| IBIS file stm32f303x6x8_334_lqfp64.ibs
[IBIS ver] 4.2
[File name] stm32f303x6x8_334_lqfp64.ibs
[File Rev] 1
[Date]  29-09-2025
[Source] Data Created at STMicroelectronics
[Notes]  File originated from ELDO simulations.
[Disclaimer]  This information is for modeling purpose only and is
   not guaranted. The information is subject to change without
   notice.
[Copyright] Copyright 2025 STMicroelectronics Inc.
|   Component stm32f303x6x8_334_lqfp64
[Component] stm32f303x6x8_334_lqfp64
[Manufacturer] STMicroelectronics
[Package]
| variable   typ   min   max
R_pkg   0.0   0.0   0.0
L_pkg   0.0H   0.0H   0.0H
C_pkg   0.0F   0.0F   0.0F
[Pin]  signal_name   model_name   R_pin   L_pin   C_pin
1 VBAT POWER 68.980E-3 4.220E-9 120.000E-15
2 PC13 io8p_sudq_tc 63.756E-3 3.679E-9 93.469E-15
3 PC14-OSC32_IN io8p_sudq_tc 59.336E-3 3.221E-9 71.020E-15
4 PC15-OSC32_OUT io8p_sudq_tc 55.719E-3 2.846E-9 52.653E-15
5 PF0-OSC_IN io8p_wsudqh_i2c_ft 52.907E-3 2.555E-9 38.367E-15
6 PF1-OSC_OUT io8p_wsudqh_i2c_ft 50.897E-3 2.347E-9 28.163E-15
7 NRST ioreset_tc_v33 49.692E-3 2.222E-9 22.041E-15
8 PC0 io8p_sudq_tc 49.290E-3 2.180E-9 20.000E-15
9 PC1 io8p_sudq_tc 49.290E-3 2.180E-9 20.000E-15
10 PC2 io8p_sudq_tc 49.692E-3 2.222E-9 22.041E-15
11 PC3 io8p_sudq_tc 50.897E-3 2.347E-9 28.163E-15
12 VSSA GND 52.907E-3 2.555E-9 38.367E-15
13 VDDA POWER 55.719E-3 2.846E-9 52.653E-15
14 PA0 io8p_sudq_tc 59.336E-3 3.221E-9 71.020E-15
15 PA1 io8p_sudq_tc 63.756E-3 3.679E-9 93.469E-15
16 PA2 io8p_sudq_tc 68.980E-3 4.220E-9 120.000E-15
17 PA3 io8p_sudq_tc 68.980E-3 4.220E-9 120.000E-15
18 VSS GND 63.756E-3 3.679E-9 93.469E-15
19 VDD POWER 59.336E-3 3.221E-9 71.020E-15
20 PA4 io8p_sudq_tc 55.719E-3 2.846E-9 52.653E-15
21 PA5 io8p_sudq_tc 52.907E-3 2.555E-9 38.367E-15
22 PA6 io8p_sudq_tc 50.897E-3 2.347E-9 28.163E-15
23 PA7 io8p_sudq_tc 49.692E-3 2.222E-9 22.041E-15
24 PC4 io8p_sudq_tc 49.290E-3 2.180E-9 20.000E-15
25 PC5 io8p_sudq_tc 49.290E-3 2.180E-9 20.000E-15
26 PB0 io8p_sudq_tc 49.692E-3 2.222E-9 22.041E-15
27 PB1 io8p_sudq_tc 50.897E-3 2.347E-9 28.163E-15
28 PB2 io8p_sudq_tc 52.907E-3 2.555E-9 38.367E-15
29 PB10 io8p_sudq_tc 55.719E-3 2.846E-9 52.653E-15
30 PB11 io8p_sudq_tc 59.336E-3 3.221E-9 71.020E-15
31 VSS GND 63.756E-3 3.679E-9 93.469E-15
32 VDD POWER 68.980E-3 4.220E-9 120.000E-15
33 PB12 io8p_sudq_tc 68.980E-3 4.220E-9 120.000E-15
34 PB13 io8p_sudq_tc 63.756E-3 3.679E-9 93.469E-15
35 PB14 io8p_sudq_tc 59.336E-3 3.221E-9 71.020E-15
36 PB15 io8p_sudq_tc 55.719E-3 2.846E-9 52.653E-15
37 PC6 io8p_sudq_ft 52.907E-3 2.555E-9 38.367E-15
38 PC7 io8p_sudq_ft 50.897E-3 2.347E-9 28.163E-15
39 PC8 io8p_sudq_ft 49.692E-3 2.222E-9 22.041E-15
40 PC9 io8p_wsudqh_i2c_ft 49.290E-3 2.180E-9 20.000E-15
41 PA8 io8p_wsudqh_i2c_ft 49.290E-3 2.180E-9 20.000E-15
42 PA9 io8p_wsudqh_i2c_ft 49.692E-3 2.222E-9 22.041E-15
43 PA10 io8p_wsudqh_i2c_ft 50.897E-3 2.347E-9 28.163E-15
44 PA11 io8usb_lv_ft 52.907E-3 2.555E-9 38.367E-15
45 PA12 io8usb_lv_ft 55.719E-3 2.846E-9 52.653E-15
46 PA13 io8p_wsudqh_i2c_ft 59.336E-3 3.221E-9 71.020E-15
47 VSS GND 63.756E-3 3.679E-9 93.469E-15
48 VDD POWER 68.980E-3 4.220E-9 120.000E-15
49 PA14 io8p_wsudqh_i2c_ft 68.980E-3 4.220E-9 120.000E-15
50 PA15 io8p_wsudqh_i2c_ft 63.756E-3 3.679E-9 93.469E-15
51 PC10 io8p_sudq_ft 59.336E-3 3.221E-9 71.020E-15
52 PC11 io8p_sudq_ft 55.719E-3 2.846E-9 52.653E-15
53 PC12 io8p_sudq_ft 52.907E-3 2.555E-9 38.367E-15
54 PD2 io8p_sudq_ft 50.897E-3 2.347E-9 28.163E-15
55 PB3 io8p_sudq_ft 49.692E-3 2.222E-9 22.041E-15
56 PB4 io8p_sudq_ft 49.290E-3 2.180E-9 20.000E-15
57 PB5 io8p_wsudqh_i2c_ft 49.290E-3 2.180E-9 20.000E-15
58 PB6 io8p_wsudqh_i2c_ft 49.692E-3 2.222E-9 22.041E-15
59 PB7 io8p_wsudqh_i2c_ft 50.897E-3 2.347E-9 28.163E-15
60 BOOT0 vpp_test_hv 52.907E-3 2.555E-9 38.367E-15
61 PB8 io8p_wsudqh_i2c_ft 55.719E-3 2.846E-9 52.653E-15
62 PB9 io8p_wsudqh_i2c_ft 59.336E-3 3.221E-9 71.020E-15
63 VSS GND 63.756E-3 3.679E-9 93.469E-15
64 VDD POWER 68.980E-3 4.220E-9 120.000E-15
[Diff Pin]   inv_pin   vdiff   tdelay_typ  tdelay_min  tdelay_max
44 45 200mV   NA   NA   NA
[Model Selector] io8p_sudq_ft
io8p01_sudq_ft_pd_lv  "SPEED01 2P0V, PD=40kOhm"
io8p01_sudq_ft_pu_lv  "SPEED01 2P0V, PU=40kOhm"
io8p01_sudq_ft_lv  "SPEED01 2P0V"
io8p10_sudq_ft_pd_lv  "SPEED10 2P0V, PD=40kOhm"
io8p10_sudq_ft_pu_lv  "SPEED10 2P0V, PU=40kOhm"
io8p10_sudq_ft_lv  "SPEED10 2P0V"
io8p11_sudq_ft_pd_lv  "SPEED11 2P0V, PD=40kOhm"
io8p11_sudq_ft_pu_lv  "SPEED11 2P0V, PU=40kOhm"
io8p11_sudq_ft_lv  "SPEED11 2P0V"
io8p01_sudq_ft_pd  "SPEED01, PD=40kOhm"
io8p01_sudq_ft_pu  "SPEED01, PU=40kOhm"
io8p01_sudq_ft  "SPEED01"
io8p10_sudq_ft_pd  "SPEED10, PD=40kOhm"
io8p10_sudq_ft_pu  "SPEED10, PU=40kOhm"
io8p10_sudq_ft  "SPEED10"
io8p11_sudq_ft_pd  "SPEED11, PD=40kOhm"
io8p11_sudq_ft_pu  "SPEED11, PU=40kOhm"
io8p11_sudq_ft  "SPEED11"
[Model Selector] io8p_sudq_tc
io8p01_sudq_tc_pd_lv  "SPEED01 2P0V, PD=40kOhm"
io8p01_sudq_tc_pu_lv  "SPEED01 2P0V, PU=40kOhm"
io8p01_sudq_tc_lv  "SPEED01 2P0V"
io8p10_sudq_tc_pd_lv  "SPEED10 2P0V, PD=40kOhm"
io8p10_sudq_tc_pu_lv  "SPEED10 2P0V, PU=40kOhm"
io8p10_sudq_tc_lv  "SPEED10 2P0V"
io8p11_sudq_tc_pd_lv  "SPEED11 2P0V, PD=40kOhm"
io8p11_sudq_tc_pu_lv  "SPEED11 2P0V, PU=40kOhm"
io8p11_sudq_tc_lv  "SPEED11 2P0V"
io8p01_sudq_tc_pd  "SPEED01, PD=40kOhm"
io8p01_sudq_tc_pu  "SPEED01, PU=40kOhm"
io8p01_sudq_tc  "SPEED01"
io8p10_sudq_tc_pd  "SPEED10, PD=40kOhm"
io8p10_sudq_tc_pu  "SPEED10, PU=40kOhm"
io8p10_sudq_tc  "SPEED10"
io8p11_sudq_tc_pd  "SPEED11, PD=40kOhm"
io8p11_sudq_tc_pu  "SPEED11, PU=40kOhm"
io8p11_sudq_tc  "SPEED11"
[Model Selector] io8p_wsudqh_i2c_ft
io8p_wsudqh_i2c_ft_lv_pd  "General purpose IO with I2C capability on. 5V tolerant. 1.8V range with pull down"
io8p_wsudqh_i2c_ft_lv_pu  "General purpose IO with I2C capability on. 5V tolerant. 1.8V range with pull up"
io8p_wsudqh_i2c_ft_lv  "General purpose IO with I2C capability on. 5V tolerant. 1.8V range"
io8p_wsudqh_i2c_ft_pd  "General purpose IO with I2C capability on. 5V tolerant. 3.3V range with pull down"
io8p_wsudqh_i2c_ft_pu  "General purpose IO with I2C capability on. 5V tolerant. 3.3V range with pull up"
io8p_wsudqh_i2c_ft_i2c  "General purpose IO with I2C capability on. 5V tolerant. 3.3V range"
[Model Selector] io8usb_lv_ft
io8usb_dpdn_lv_ft_pd  "FS USB DP/DN IO + PD=40kOhm"
io8usb_dpdn_lv_ft_pu  "FS USB DP/DN IO + PU=40kOhm"
io8usb_dpdn_lv_ft  "FS USB DP/DN IO"
io8p01_lv_ft_pd_lv  "SPEED01 2P0V, PD=40kOhm"
io8p01_lv_ft_pu_lv  "SPEED01 2P0V, PU=40kOhm"
io8p01_lv_ft_lv  "SPEED01 2P0V"
io8p10_lv_ft_pd_lv  "SPEED10 2P0V, PD=40kOhm"
io8p10_lv_ft_pu_lv  "SPEED10 2P0V, PU=40kOhm"
io8p10_lv_ft_lv  "SPEED10 2P0V"
io8p11_lv_ft_pd_lv  "SPEED11 2P0V, PD=40kOhm"
io8p11_lv_ft_pu_lv  "SPEED11 2P0V, PU=40kOhm"
io8p11_lv_ft_lv  "SPEED11 2P0V"
io8p01_lv_ft_pd  "SPEED01, PD=40kOhm"
io8p01_lv_ft_pu  "SPEED01, PU=40kOhm"
io8p01_lv_ft  "SPEED01"
io8p10_lv_ft_pd  "SPEED10, PD=40kOhm"
io8p10_lv_ft_pu  "SPEED10, PU=40kOhm"
io8p10_lv_ft  "SPEED10"
io8p11_lv_ft_pd  "SPEED11, PD=40kOhm"
io8p11_lv_ft_pu  "SPEED11, PU=40kOhm"
io8p11_lv_ft  "SPEED11"
[Model Selector] ioreset_tc_v33
ioreset_tc_v33_pu_lv  "IORESET 2V + PU=40kOhm"
ioreset_tc_v33_nopu_lv  "IORESET 2V"
ioreset_tc_v33_pu  "IORESET + PU=40kOhm"
ioreset_tc_v33_nopu  "IORESET"
[Model Selector] vpp_test_hv
vpp_test_hv_3p3  "Input Buffer"
vpp_test_hv_2p4  "Input Buffer 2P0V"
| Models and submodels in the file (69): io8p01_sudq_ft_pd_lv (I/O), io8p01_sudq_ft_pu_lv (I/O), io8p01_sudq_ft_lv (I/O), io8p10_sudq_ft_pd_lv (I/O), io8p10_sudq_ft_pu_lv (I/O), io8p10_sudq_ft_lv (I/O), io8p11_sudq_ft_pd_lv (I/O), io8p11_sudq_ft_pu_lv (I/O), io8p11_sudq_ft_lv (I/O), io8p01_sudq_ft_pd (I/O), io8p01_sudq_ft_pu (I/O), io8p01_sudq_ft (I/O), io8p10_sudq_ft_pd (I/O), io8p10_sudq_ft_pu (I/O), io8p10_sudq_ft (I/O), io8p11_sudq_ft_pd (I/O), io8p11_sudq_ft_pu (I/O), io8p11_sudq_ft (I/O), io8p01_sudq_tc_pd_lv (I/O), io8p01_sudq_tc_pu_lv (I/O), io8p01_sudq_tc_lv (I/O), io8p10_sudq_tc_pd_lv (I/O), io8p10_sudq_tc_pu_lv (I/O), io8p10_sudq_tc_lv (I/O), io8p11_sudq_tc_pd_lv (I/O), io8p11_sudq_tc_pu_lv (I/O), io8p11_sudq_tc_lv (I/O), io8p01_sudq_tc_pd (I/O), io8p01_sudq_tc_pu (I/O), io8p01_sudq_tc (I/O), io8p10_sudq_tc_pd (I/O), io8p10_sudq_tc_pu (I/O), io8p10_sudq_tc (I/O), io8p11_sudq_tc_pd (I/O), io8p11_sudq_tc_pu (I/O), io8p11_sudq_tc (I/O), io8p_wsudqh_i2c_ft_lv_pd (I/O), io8p_wsudqh_i2c_ft_lv_pu (I/O), io8p_wsudqh_i2c_ft_lv (I/O), io8p_wsudqh_i2c_ft_pd (I/O), io8p_wsudqh_i2c_ft_pu (I/O), io8p_wsudqh_i2c_ft_i2c (I/O), io8usb_dpdn_lv_ft_pd (I/O), io8usb_dpdn_lv_ft_pu (I/O), io8usb_dpdn_lv_ft (I/O), io8p01_lv_ft_pd_lv (I/O), io8p01_lv_ft_pu_lv (I/O), io8p01_lv_ft_lv (I/O), io8p10_lv_ft_pd_lv (I/O), io8p10_lv_ft_pu_lv (I/O), io8p10_lv_ft_lv (I/O), io8p11_lv_ft_pd_lv (I/O), io8p11_lv_ft_pu_lv (I/O), io8p11_lv_ft_lv (I/O), io8p01_lv_ft_pd (I/O), io8p01_lv_ft_pu (I/O), io8p01_lv_ft (I/O), io8p10_lv_ft_pd (I/O), io8p10_lv_ft_pu (I/O), io8p10_lv_ft (I/O), io8p11_lv_ft_pd (I/O), io8p11_lv_ft_pu (I/O), io8p11_lv_ft (I/O), ioreset_tc_v33_pu_lv (I/O_open_drain), ioreset_tc_v33_nopu_lv (I/O_open_drain), ioreset_tc_v33_pu (I/O_open_drain), ioreset_tc_v33_nopu (I/O_open_drain), vpp_test_hv_2p4 (Input), vpp_test_hv_3p3 (Input)
